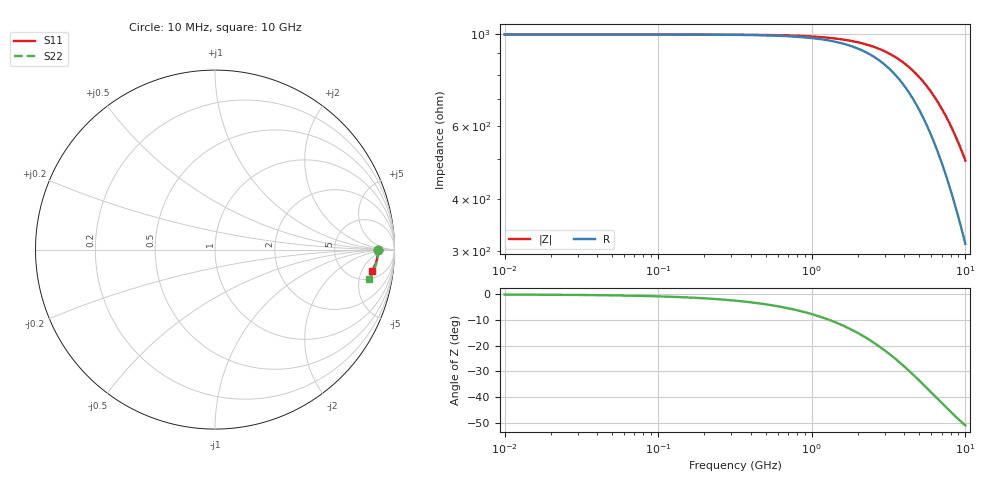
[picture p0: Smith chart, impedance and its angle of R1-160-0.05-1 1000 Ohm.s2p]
!version-1
!date-03.2021
# MHz S RI R 50
!Freq ReS11 ImS11 ReS21 ImS21 ReS12 ImS12 ReS22 ImS22
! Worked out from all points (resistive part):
!   501 points, 10 MHz to 10 GHz, reference 50 ohm
!   read as one part in series: R = 1 kohm at 50 MHz
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10  0.9091 -0.000112  0.0909 0.00011  0.0909 0.00011  0.9091 -0.000151
410  0.909 -0.00458  0.091 0.0045  0.091 0.0045  0.909 -0.0062
610  0.909 -0.00682  0.091 0.0067  0.091 0.0067  0.9089 -0.00923
830  0.9089 -0.00927  0.0911 0.00911  0.0911 0.00911  0.9088 -0.0126
1250  0.9086 -0.014  0.0914 0.0137  0.0914 0.0137  0.9085 -0.0189
1470  0.9085 -0.0164  0.0916 0.0162  0.0916 0.0162  0.9082 -0.0223
1690  0.9083 -0.0189  0.0919 0.0186  0.0919 0.0186  0.9079 -0.0256
2090  0.9079 -0.0234  0.0924 0.023  0.0924 0.023  0.9073 -0.0317
2490  0.9073 -0.0279  0.093 0.0275  0.093 0.0275  0.9066 -0.0379
2910  0.9067 -0.0326  0.0938 0.0321  0.0938 0.0321  0.9056 -0.0443
3350  0.9059 -0.0376  0.0948 0.0371  0.0948 0.0371  0.9045 -0.0512
3730  0.9051 -0.042  0.0957 0.0414  0.0957 0.0414  0.9034 -0.0571
4130  0.9041 -0.0465  0.0968 0.0459  0.0968 0.0459  0.902 -0.0634
4550  0.903 -0.0514  0.0981 0.0507  0.0981 0.0507  0.9005 -0.07
5010  0.9017 -0.0567  0.0998 0.0561  0.0998 0.0561  0.8985 -0.0774
5790  0.8991 -0.0658  0.1029 0.0652  0.1029 0.0652  0.8948 -0.0901
6670  0.8955 -0.0762  0.1072 0.0757  0.1072 0.0757  0.8896 -0.1048
7530  0.8914 -0.0865  0.1121 0.0863  0.1121 0.0863  0.8837 -0.1195
8350  0.8868 -0.0965  0.1177 0.0966  0.1177 0.0966  0.877 -0.1339
9170  0.8815 -0.1066  0.1241 0.1072  0.1241 0.1072  0.8692 -0.1487
9950  0.8757 -0.1164  0.1312 0.1175  0.1312 0.1175  0.8606 -0.1633
10000  0.8753 -0.117  0.1317 0.1182  0.1317 0.1182  0.86 -0.1642
